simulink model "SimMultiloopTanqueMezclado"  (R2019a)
settings: Solver=VariableStepAuto  StartTime=0.0  StopTime=18  RelTol=1e-5  AbsTol=1e-5
PreLoadFcn:
  | load ModeloTanqueLin
  | TanqueMezcladoLin.OutputDelay=[0.15;0];
  | s=tf('s');
  | Gact=1/(0.02*s+1);
  | PIDnivel=3.5+6/s;
  | PIDconc_qb=-(3.75+12/s);
  | PIDconc_qa=(11+33/s);
libraries: cstblocks x13, simulink x2

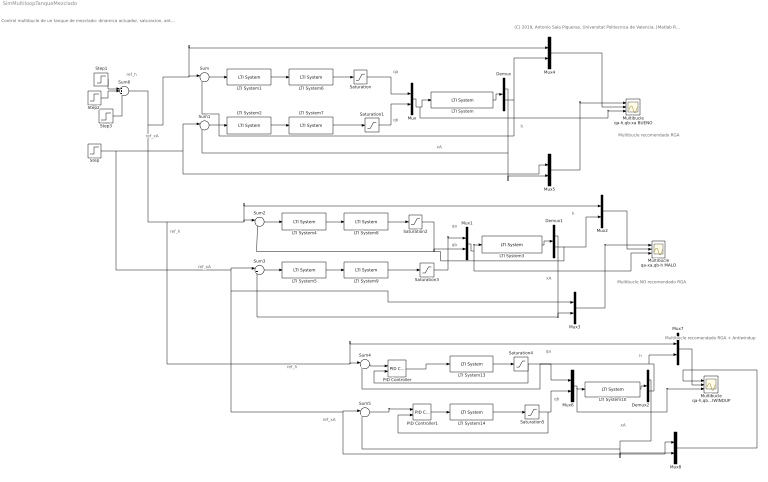
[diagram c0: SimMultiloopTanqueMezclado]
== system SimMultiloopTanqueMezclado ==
  note: (C) 2019, Antonio Sala Piqueras, Universitat Politecnica de Valencia. [Matlab R2019a]
  note: Control multibucle de un tanque de mezclado: dinamica actuador, saturacion, antiwindup
  note: Multibucle recomendado RGA
  note: ref_xA
  note: ref_h
  note: h
  note: xA
  note: qb
  note: qa
  note: xA
  note: qb
  note: h
  note: qa
  note: ref_h
  note: ref_xA
  note: h
  note: ref_h
  note: xA
  note: qb
  note: qa
  note: ref_xA
  note: Multibucle NO recomendado RGA
  note: Multibucle recomendado RGA + Antiwindup
  Demux : Demux  Outputs=2
  Demux1 : Demux  Outputs=2
  Demux2 : Demux  Outputs=2
  LTI System : cstblocks/LTI System  sys=TanqueMezcladoLin  IC=[]
  LTI System1 : cstblocks/LTI System  sys=PIDnivel  IC=[]
  LTI System10 : cstblocks/LTI System  sys=TanqueMezcladoLin  IC=[]
  LTI System{6..9,13..14} (6 alike) : cstblocks/LTI System  sys=Gact  IC=[]
  LTI System2 : cstblocks/LTI System  sys=PIDconc_qb  IC=[]
  LTI System3 : cstblocks/LTI System  sys=TanqueMezcladoLin  IC=[]
  LTI System4 : cstblocks/LTI System  sys=PIDnivel  IC=[]
  LTI System5 : cstblocks/LTI System  sys=PIDconc_qa  IC=[]
  Multibucle qa-h,qb-xa BUENO : Scope  NumInputPorts=3
  Multibucle qa-h,qb-xa1 ANTIWINDUP : Scope  NumInputPorts=3
  Multibucle qa-xa,qb-h MALO : Scope  NumInputPorts=3
  Mux{,1..8} (9 alike) : Mux  Inputs=2
  PID Controller : simulink/Continuous/PID Controller  Controller=PID  Form=Parallel  TimeDomain=Continuous-time  SampleTime=-1  IntegratorMethod=Forward Euler  FilterMethod=Forward Euler  ControllerParametersSource=internal  P=3.5  I=6  D=0  UseFilter=on  N=100  TunerSelectOption=Transfer Function Based (PID Tuner App)  InitialConditionSource=internal  InitialConditionForIntegrator=0  InitialConditionForFilter=0  DifferentiatorICPrevScaledInput=0  ExternalReset=none  TrackingMode=on  Kt=0.5  LimitOutput=off  UpperSaturationLimit=inf  LowerSaturationLimit=-inf  LinearizeAsGain=on  AntiWindupMode=none  Kb=1  POutMin=[]  POutMax=[]  IOutMin=[]  IOutMax=[]  DOutMin=[]  DOutMax=[]  NOutMin=[]  NOutMax=[]  SumOutMin=[]  SumOutMax=[]  SaturationOutMin=[]  SaturationOutMax=[]  PParamMin=[]  PParamMax=[]  IParamMin=[]  IParamMax=[]  DParamMin=[]  DParamMax=[]  NParamMin=[]  NParamMax=[]  KbParamMin=[]  KbParamMax=[]  KtParamMin=[]  KtParamMax=[]  KbOutMin=[]  KbOutMax=[]  KtOutMin=[]  KtOutMax=[]  IntegratorOutMin=[]  IntegratorOutMax=[]  FilterOutMin=[]  FilterOutMax=[]  SumI1OutMin=[]  SumI1OutMax=[]  SumI2OutMin=[]  SumI2OutMax=[]  SumI3OutMin=[]  SumI3OutMax=[]  SumI4OutMin=[]  SumI4OutMax=[]  SumDOutMin=[]  SumDOutMax=[]  DifferentiatorOutMin=[]  DifferentiatorOutMax=[]  FilterDiffOutCoefMin=[]  FilterDiffOutCoefMax=[]  ReciprocalOutMin=[]  ReciprocalOutMax=[]  SumDenOutMin=[]  SumDenOutMax=[]  SumNumOutMin=[]  SumNumOutMax=[]  DivideOutMin=[]  DivideOutMax=[]  IntegratorContinuousStateAttributes=''  IntegratorStateMustResolveToSignalObject=off  IntegratorRTWStateStorageClass=Auto  FilterContinuousStateAttributes=''  FilterStateMustResolveToSignalObject=off  FilterRTWStateStorageClass=Auto  ParallelPVariant=InternalParameters  IdealPVariant=Disabled  IVariant=InternalParameters  DVariant=InternalParameters  IntegratorVariant=Continuous  SatVariant=Disabled  AWVariant=Passthrough  PCopyVariant=Disabled  TRVariant=Enabled  FdbkBlocksVariant=Forward  IdealPFdbkVariant=Disabled  SatFdbkVariant=Disabled  DerivativeFilterVariant=ContFilter  NVariant=InternalParameters  NCopyVariant=Disabled  FilterICVariant=InternalICsFilter  IntegratorICVariant=InternalICs  ExternalResetVariant=Disabled  TRSumVariant=TrackingMode  SumFdbkVariant=Disabled  SumVariant=Sum_PID
  PID Controller1 : simulink/Continuous/PID Controller  Controller=PID  Form=Parallel  TimeDomain=Continuous-time  SampleTime=-1  IntegratorMethod=Forward Euler  FilterMethod=Forward Euler  ControllerParametersSource=internal  P=-3.75  I=-12  D=0  UseFilter=on  N=100  TunerSelectOption=Transfer Function Based (PID Tuner App)  InitialConditionSource=internal  InitialConditionForIntegrator=0  InitialConditionForFilter=0  DifferentiatorICPrevScaledInput=0  ExternalReset=none  TrackingMode=on  Kt=0.5  LimitOutput=off  UpperSaturationLimit=inf  LowerSaturationLimit=-inf  LinearizeAsGain=on  AntiWindupMode=none  Kb=1  POutMin=[]  POutMax=[]  IOutMin=[]  IOutMax=[]  DOutMin=[]  DOutMax=[]  NOutMin=[]  NOutMax=[]  SumOutMin=[]  SumOutMax=[]  SaturationOutMin=[]  SaturationOutMax=[]  PParamMin=[]  PParamMax=[]  IParamMin=[]  IParamMax=[]  DParamMin=[]  DParamMax=[]  NParamMin=[]  NParamMax=[]  KbParamMin=[]  KbParamMax=[]  KtParamMin=[]  KtParamMax=[]  KbOutMin=[]  KbOutMax=[]  KtOutMin=[]  KtOutMax=[]  IntegratorOutMin=[]  IntegratorOutMax=[]  FilterOutMin=[]  FilterOutMax=[]  SumI1OutMin=[]  SumI1OutMax=[]  SumI2OutMin=[]  SumI2OutMax=[]  SumI3OutMin=[]  SumI3OutMax=[]  SumI4OutMin=[]  SumI4OutMax=[]  SumDOutMin=[]  SumDOutMax=[]  DifferentiatorOutMin=[]  DifferentiatorOutMax=[]  FilterDiffOutCoefMin=[]  FilterDiffOutCoefMax=[]  ReciprocalOutMin=[]  ReciprocalOutMax=[]  SumDenOutMin=[]  SumDenOutMax=[]  SumNumOutMin=[]  SumNumOutMax=[]  DivideOutMin=[]  DivideOutMax=[]  IntegratorContinuousStateAttributes=''  IntegratorStateMustResolveToSignalObject=off  IntegratorRTWStateStorageClass=Auto  FilterContinuousStateAttributes=''  FilterStateMustResolveToSignalObject=off  FilterRTWStateStorageClass=Auto  ParallelPVariant=InternalParameters  IdealPVariant=Disabled  IVariant=InternalParameters  DVariant=InternalParameters  IntegratorVariant=Continuous  SatVariant=Disabled  AWVariant=Passthrough  PCopyVariant=Disabled  TRVariant=Enabled  FdbkBlocksVariant=Forward  IdealPFdbkVariant=Disabled  SatFdbkVariant=Disabled  DerivativeFilterVariant=ContFilter  NVariant=InternalParameters  NCopyVariant=Disabled  FilterICVariant=InternalICsFilter  IntegratorICVariant=InternalICs  ExternalResetVariant=Disabled  TRSumVariant=TrackingMode  SumFdbkVariant=Disabled  SumVariant=Sum_PID
  Saturation{,1..5} (6 alike) : Saturate  UpperLimit=2  LowerLimit=-2
  Step : Step  After=.2  SampleTime=0
  Step1 : Step  Time=4  After=0.4  SampleTime=0
  Step2 : Step  Time=7.5  After=0.8  SampleTime=0
  Step3 : Step  Time=11  After=-1.75  SampleTime=0
  Sum{,1..5} (6 alike) : Sum  Inputs=|+-
  Sum6 : Sum  Inputs=+++
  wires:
  LTI System/1 -> Demux/1
  Mux/1 -> Multibucle qa-h,qb-xa BUENO/3, LTI System/1
  Sum/1 -> LTI System1/1
  LTI System2/1 -> LTI System7/1
  Demux/2 -> Sum/2, Mux4/2
  LTI System1/1 -> LTI System6/1
  Sum1/1 -> LTI System2/1
  Step1/1 -> Sum6/1
  Step2/1 -> Sum6/2
  LTI System6/1 -> Saturation/1
  Saturation/1 -> Mux/1
  LTI System7/1 -> Saturation1/1
  Saturation1/1 -> Mux/2
  Mux5/1 -> Multibucle qa-h,qb-xa BUENO/1
  Step3/1 -> Sum6/3
  LTI System9/1 -> Saturation3/1
  LTI System8/1 -> Saturation2/1
  LTI System3/1 -> Demux1/1
  Sum3/1 -> LTI System5/1
  Mux3/1 -> Multibucle qa-xa,qb-h MALO/1
  LTI System4/1 -> LTI System8/1
  Mux1/1 -> Multibucle qa-xa,qb-h MALO/3, LTI System3/1
  LTI System5/1 -> LTI System9/1
  Sum2/1 -> LTI System4/1
  Demux1/2 -> Sum2/2, Mux2/2
  Demux1/1 -> Mux3/2, Sum3/2
  Saturation3/1 -> Mux1/1
  Saturation2/1 -> Mux1/2
  Saturation4/1 -> PID Controller/2, Mux6/1
  Saturation5/1 -> PID Controller1/2, Mux6/2
  Mux8/1 -> Multibucle qa-h,qb-xa1 ANTIWINDUP/1
  Sum6/1 -> Mux7/1, Sum4/1, Mux2/1, Sum2/1, Mux4/1, Sum/1
  LTI System14/1 -> Saturation5/1
  Sum5/1 -> PID Controller1/1
  Step/1 -> Sum1/1, Mux5/1, Mux3/1, Mux8/1, Sum5/1, Sum3/1
  Demux2/2 -> Mux7/2, Sum4/2
  Demux2/1 -> Mux8/2, Sum5/2
  Sum4/1 -> PID Controller/1
  LTI System13/1 -> Saturation4/1
  LTI System10/1 -> Demux2/1
  PID Controller1/1 -> LTI System14/1
  Mux6/1 -> Multibucle qa-h,qb-xa1 ANTIWINDUP/3, LTI System10/1
  PID Controller/1 -> LTI System13/1
  Demux/1 -> Mux5/2, Sum1/2
  Mux4/1 -> Multibucle qa-h,qb-xa BUENO/2
  Mux2/1 -> Multibucle qa-xa,qb-h MALO/2
  Mux7/1 -> Multibucle qa-h,qb-xa1 ANTIWINDUP/2
